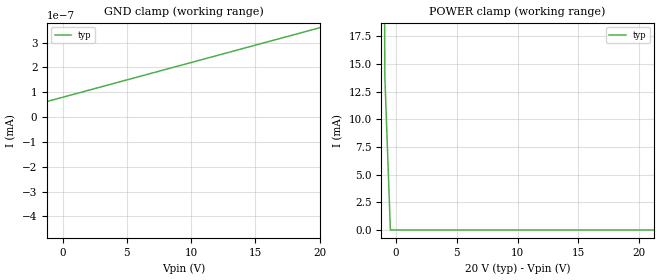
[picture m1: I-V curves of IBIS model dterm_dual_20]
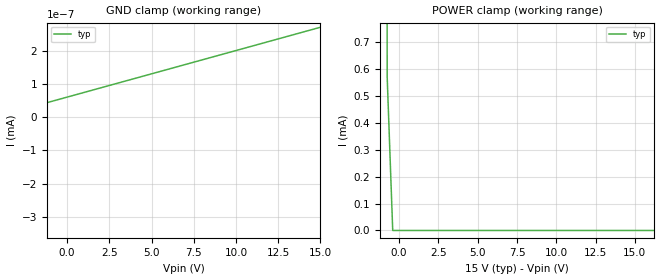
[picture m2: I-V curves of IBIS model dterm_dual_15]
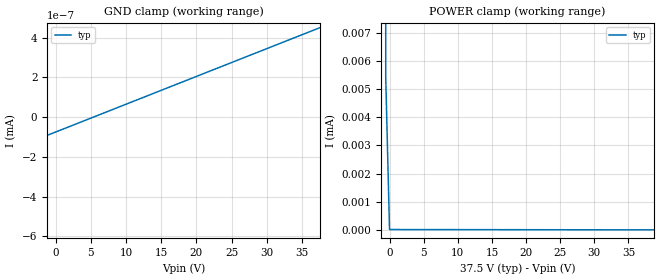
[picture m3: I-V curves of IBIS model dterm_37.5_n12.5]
|Texas Instruments Incorporated
|tmux7612, 4 Data Lane 1:1 Switch (4-Channel, 1:1 Analog Switch)
[IBIS Ver]   4.1
[File name]   tmux7612ca.ibs
[Date]   06/13/23
[File Rev]   1.0
[Source]
| Texas Instruments Incorporated.
| ASC-INT-MUX
| 12500 TI Blvd
| Dallas, TX - 75243
[Notes]   Revision History:
| Rev 1.0: 06/13/23
| - Initial version of the model
| - Model generated from simulations in SPECTRE
| - C_comp although listed in numerical order of value are
|   obtained from varying PVT conditions. For PVT conditions for
|   each specific value refer the buffer description under
|   respective [Model]. IBIS model user is responsible for using
|   appropriate C_comp to simulate for Signal Integrity.
[Disclaimer]
| This model is designed as an aid for customers of Texas Instruments.
| TI and its licensors and suppliers make no warranties, either expressed
| or implied, with respect to this  model, including the warranties of
| merchantability or fitness for a particular purpose. The model is
| provided solely on an "as is" basis. The entire risk as to its quality
| and performance is with the customer.
| This model is subject to change without notice. Texas Instruments
| Incorporated is not responsible for updating this model.
[Copyright]
(C) Copyright 2023 Texas Instruments Incorporated.All rights reserved.
|  Component TMUX7612PW 16-pin - PW package
|  Part # TMUX7612PW
[Component]   TMUX7612PW
[Manufacturer]  TI
[Package]
|   typ   min   max
R_pkg   0.0668   NA   NA
L_pkg   2.1992nH   NA   NA
C_pkg   0.2884pF   NA   NA
[Pin]   signal_name   model_name
   1   SEL1   inbuf
   2   D1   dterm
   3   S1   sterm
   4   VSS   power
   5   GND   gnd
   6   S4   sterm
   7   D4   dterm
   8   SEL4   inbuf
   9   SEL3   inbuf
   10   D3   dterm
   11   S3   sterm
   12   NC   nc
   13   VDD   power
   14   S2   sterm
   15   D2   dterm
   16   SEL2   inbuf
[Series Switch Groups]
On 1 /
On 2 /
On 3 /
On 4 /
Off 1 2 3 4 /
[Series Pin Mapping]  pin_2 model_name function_table_group
   2   3   switch_dual_20   1
   6   7   switch_dual_20   1
  10  11   switch_dual_20   1
  14  15   switch_dual_20   1
|   2   3   switch_dual_15   1
|   6   7   switch_dual_15   1
|  10  11   switch_dual_15   1
|  14  15   switch_dual_15   1
|   2   3  switch_37.5_n12.5   1
|   6   7  switch_37.5_n12.5   1
|  10  11  switch_37.5_n12.5   1
|  14  15  switch_37.5_n12.5   1
|   2   3   switch_12   1
|   6   7   switch_12   1
|  10  11   switch_12   1
|  14  15   switch_12   1
|  Component TMUX7612RUM 16-pin - RUM package
|  Part # TMUX7612RUM
[Component]   TMUX7612RUM
[Manufacturer]  TI
[Package]
|   typ   min   max
R_pkg   0.067   NA   NA
L_pkg   0.0001nH   NA   NA
C_pkg   0.144pF   NA   NA
[Pin]   signal_name   model_name
   1   S1   sterm
   2   VSS   power
   3   GND   gnd
   4   S4   sterm
   5   D4   dterm
   6   SEL4   inbuf
   7   SEL3   inbuf
   8   D3   dterm
   9   S3   sterm
   10   NC   nc
   11   VDD   power
   12   S2   sterm
   13   D2   dterm
   14   SEL2   inbuf
   15   SEL1   inbuf
   16   D1   dterm
[Series Switch Groups]
On 1 /
On 2 /
On 3 /
On 4 /
Off 1 2 3 4 /
[Series Pin Mapping]  pin_2 model_name function_table_group
|  16   1   switch_dual_20   1
|   4   5   switch_dual_20   1
|   8   9   switch_dual_20   1
|  12  13   switch_dual_20   1
|  16   1   switch_dual_15   1
|  4   5   switch_dual_15   1
|  8   9   switch_dual_15   1
| 12  13   switch_dual_15   1
|  16   1  switch_37.5_n12.5   1
|   4   5  switch_37.5_n12.5   1
|   8   9  switch_37.5_n12.5   1
|  12  13  switch_37.5_n12.5   1
  16   1  switch_12   1
   4   5  switch_12   1
   8   9  switch_12   1
  12  13  switch_12   1
[Model Selector] dterm
dterm_dual_20 Use for operation at +/-20V
dterm_dual_15 Use for operation at +/-15V
dterm_37.5_n12.5 Use for operation at 37V
dterm_12 Use for operation at 12V
[Model Selector] sterm
sterm_dual_20 Use for operation at +/-20V
sterm_dual_15 Use for operation at +/-15V
sterm_37.5_n12.5 Use for operation at 37V
sterm_12 Use for operation at 12V
[Model Selector] inbuf
inbuf_dual_20 Use for operation at +/-20V
inbuf_dual_15 Use for operation at +/-15V
inbuf_37.5_n12.5 Use for operation at +37V/-12.5V
inbuf_12 Use for operation at 12V
| switch_dual_20
[Model]   switch_dual_20
Model_type   Series_switch
|   typ   min   max
C_comp   2.533030e-11   NA   NA
[Voltage Range]   20   NA   NA
[Power Clamp Reference]   20   NA   NA
[Temperature Range]   27   NA   NA
[On]
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[Off]
|   typ   min   max
[R Series]   10G   NA   NA
| switch_dual_15
[Model]   switch_dual_15
Model_type   Series_switch
|   typ   min   max
C_comp   2.533030e-11   NA   NA
[Voltage Range]   15   NA   NA
[Power Clamp Reference]   15   NA   NA
[Temperature Range]   27   NA   NA
[On]
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[Off]
|   typ   min   max
[R Series]   10G   NA   NA
| switch_37.5_n12.5
[Model]   switch_37.5_n12.5
Model_type   Series_switch
|   typ   min   max
C_comp   2.533030e-11   NA   NA
[Voltage Range]   37.5   NA   NA
[Power Clamp Reference]   37.5   NA   NA
[Temperature Range]   27   NA   NA
[On]
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[Off]
|   typ   min   max
[R Series]   10G   NA   NA
| switch_12
[Model]   switch_12
Model_type   Series_switch
|   typ   min   max
C_comp   4.014581e-11   NA   NA
[Voltage Range]   12   NA   NA
[Power Clamp Reference]   12   NA   NA
[Temperature Range]   27   NA   NA
[On]
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[Off]
|   typ   min   max
[R Series]   10G   NA   NA
| Models and submodels in the file (16): dterm_dual_20 (Terminator), dterm_dual_15 (Terminator), dterm_37.5_n12.5 (Terminator), dterm_12 (Terminator), switch_dual_20 (Series_switch), switch_dual_15 (Series_switch), switch_37.5_n12.5 (Series_switch), switch_12 (Series_switch), sterm_dual_20 (Terminator), sterm_dual_15 (Terminator), sterm_37.5_n12.5 (Terminator), sterm_12 (Terminator), inbuf_dual_20 (Input), inbuf_dual_15 (Input), inbuf_37.5_n12.5 (Input), inbuf_12 (Input)
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| dterm_dual_20
[Model]   dterm_dual_20
Model_type   Terminator
|   typ   min   max
C_comp   2.533030e-11   NA   NA
[Voltage Range]   20   NA   NA
[Temperature Range]   27   NA   NA
[Power Clamp Reference]   20   NA   NA
[GND Clamp Reference]   0   NA   NA
[GND Clamp]
|   Voltage   I(typ)   I(min)   I(max)
-25V      -2.406A    NA         NA
-20.45V   -4.99nA    NA         NA
-20V      -200pA     NA         NA
20V       360pA      NA         NA
[POWER Clamp]
|   Voltage   I(typ)   I(min)   I(max)
-5V       2.671A     NA         NA
-1.364V   132.2mA    NA         NA
-909.1mV  13.84mA    NA         NA
-454.5mV  183.5nA    NA         NA
40V       -4.294nA   NA         NA
| dterm_dual_15
[Model]   dterm_dual_15
Model_type   Terminator
|   typ   min   max
C_comp   2.533030e-11   NA   NA
[Voltage Range]   15   NA   NA
[Temperature Range]   27   NA   NA
[Power Clamp Reference]   15   NA   NA
[GND Clamp Reference]   0   NA   NA
[GND Clamp]
|   Voltage   I(typ)   I(min)   I(max)
-20V      -2.406A    NA         NA
-15.4V    -989.9pA   NA         NA
-15.05V   -150.7pA   NA         NA
15V       270pA      NA         NA
[POWER Clamp]
|   Voltage   I(typ)   I(min)   I(max)
-5V       2.668A     NA         NA
-1.111V   61.29mA    NA         NA
-757.6mV  572.1uA    NA         NA
-404mV    33.07nA    NA         NA
30V       -3.217nA   NA         NA
| dterm_37.5_n12.5
[Model]   dterm_37.5_n12.5
Model_type   Terminator
|   typ   min   max
C_comp   2.533030e-11   NA   NA
[Voltage Range]   37.5   NA   NA
[Temperature Range]   27   NA   NA
[Power Clamp Reference]   37.5   NA   NA
[GND Clamp Reference]   0   NA   NA
[GND Clamp]
|   Voltage   I(typ)   I(min)   I(max)
-17.5V    -2.406A    NA         NA
-13.06V   -161nA     NA         NA
-12.5V    -250pA     NA         NA
37.5V     450pA      NA         NA
[POWER Clamp]
|   Voltage   I(typ)   I(min)   I(max)
-5V       2.674A     NA         NA
-1.111V   61.34mA    NA         NA
-555.6mV  5.431uA    NA         NA
0V        11.38nA    NA         NA
50V       -5.372nA   NA         NA
